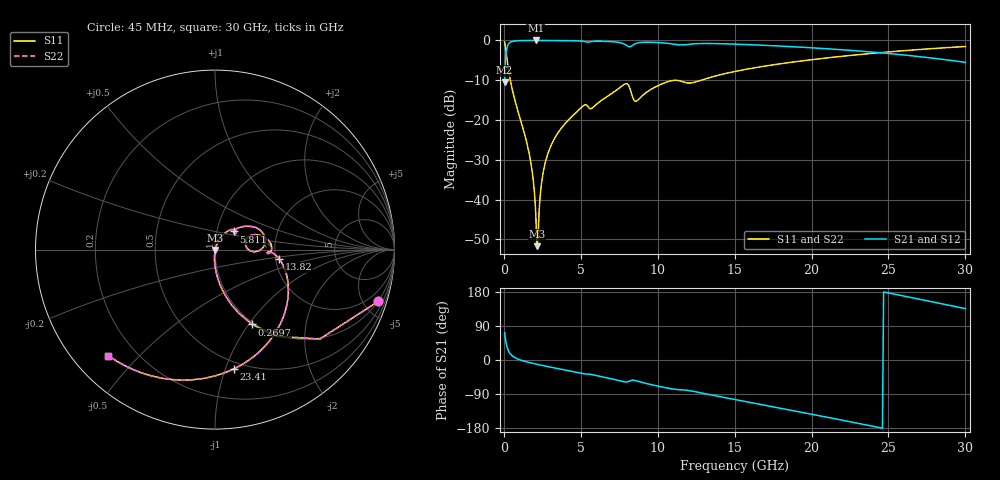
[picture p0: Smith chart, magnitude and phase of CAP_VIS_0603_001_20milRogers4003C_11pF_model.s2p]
! S-parameter model data by Modelithics Inc.  support@modelithics.com  813-866-6335  Tampa FL USA
! S-Parameter data specifications:
! Substrate: 20-mil Rogers 4003C, substrate thickness, H=0.508mm, Dielectric constant, Er=3.75
! PCB Mounting Pad Footprint: Pad width, PadW=0.90mm , Pad length, PadL=1.00mm , Pad gap, PadG (edge-to-edge)=1.00mm , Reference planes=3.0mm apart
! Created Wed Nov 18 13:26:09 2015
# hz S ma R 50
! 2 Port Network Data from SP1.SP block
! freq  magS11  angS11  magS21  angS21  magS12  angS12  magS22  angS22
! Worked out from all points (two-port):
!   401 points, 45 MHz to 30 GHz, reference 50 ohm
!   highest |S21| = -0.02 dB at 2.067 GHz (marker M1); lowest = -10.5 dB at 45 MHz (marker M2)
!   |S21| within 3 dB of the highest: 151.9 MHz to 24.19 GHz (24.04 GHz wide, 198 % of centre)
!   lowest |S11| = -51.7 dB at 2.142 GHz (marker M3), VSWR 1.01, Z = 50.1 - j0.223 ohm
!   |S11| at or under -10 dB: 416.5 MHz to 12.82 GHz (12.4 GHz wide, 187 % of centre)
!   |S22| runs from -51.7 to -0.4 dB; largest |S21 - S12| = 0
!   S11 on the Smith chart (normalised r, x): 45 MHz: 0.97, -6.32; 269.7 MHz: 0.98, -1.04; 5.811 GHz: 1.20, +0.25; 13.82 GHz: 2.09, -0.24; 23.41 GHz: 0.44, -1.07; 30 GHz: 0.10, -0.41
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4.5e7  0.9545 -17.6  0.2982 72.4  0.2982 72.4  0.9545 -17.6
2.696625e8  0.4655 -63.6  0.8844 26.3  0.8844 26.3  0.4655 -63.6
6.441e8  0.2 -81.6  0.9788 8.1  0.9788 8.1  0.2 -81.6
1.692525e9  0.03376 -94.4  0.9977 -7.1  0.9977 -7.1  0.03376 -94.4
1.917188e9  0.01689 -93.6  0.998 -9.3  0.998 -9.3  0.01689 -93.6
2.066962e9  0.006921 -86.2  0.9981 -10.6  0.9981 -10.6  0.006921 -86.2
2.14185e9  0.002607 -58.8  0.9981 -11.3  0.9981 -11.3  0.002607 -58.8
2.291625e9  0.007417 63.1  0.9979 -12.6  0.9979 -12.6  0.007417 63.1
2.4414e9  0.0159 69.2  0.9978 -13.9  0.9978 -13.9  0.0159 69.2
2.591175e9  0.02406 70.1  0.9975 -15.2  0.9975 -15.2  0.02406 70.1
2.965612e9  0.04317 68.9  0.9967 -18.3  0.9967 -18.3  0.04317 68.9
5.062462e9  0.1454 50.3  0.9777 -35.3  0.9777 -35.3  0.1454 50.3
5.811338e9  0.1455 44.2  0.9724 -39.3  0.9724 -39.3  0.1455 44.2
7.8333e9  0.2815 19.5  0.8982 -57.6  0.8982 -57.6  0.2815 19.5
8.582175e9  0.1718 10.8  0.9156 -54.7  0.9156 -54.7  0.1718 10.8
1.007992e10  0.2738 15.9  0.939 -69.5  0.939 -69.5  0.2738 15.9
1.38243e10  0.3607 -8.1  0.9115 -94.9  0.9115 -94.9  0.3607 -8.1
1.50225e10  0.4075 -16.4  0.8974 -104.4  0.8974 -104.4  0.4075 -16.4
2.003996e10  0.5736 -54.4  0.8069 -143.4  0.8069 -143.4  0.5736 -54.4
2.34099e10  0.6725 -81.0  0.7272 -170.2  0.7272 -170.2  0.6725 -81.0
2.505742e10  0.7178 -94.3  0.6828 176.5  0.6828 176.5  0.7178 -94.3
3e10  0.8378 -135.1  0.5298 135.6  0.5298 135.6  0.8378 -135.1
